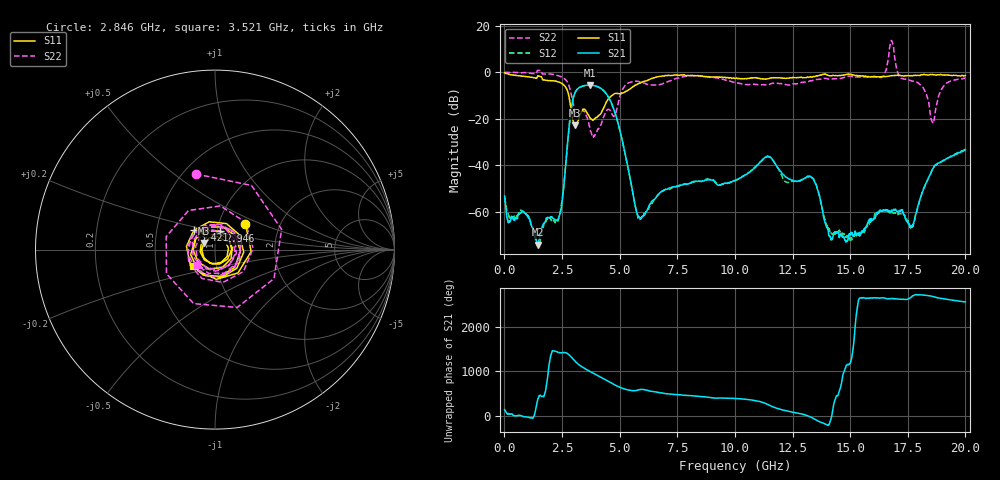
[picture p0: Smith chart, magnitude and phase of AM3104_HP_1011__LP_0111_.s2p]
!Created with skrf (http://scikit-rf.org).
# Hz S RI R 50.0
!freq ReS11 ImS11 ReS21 ImS21 ReS12 ImS12 ReS22 ImS22
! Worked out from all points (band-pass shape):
!   1601 points, 10 MHz to 20 GHz, reference 50 ohm
!   highest |S21| = -5.47 dB at 3.708 GHz (marker M1); lowest = -74.0 dB at 1.447 GHz (marker M2)
!   |S21| within 3 dB of the highest: 3.081 GHz to 4.359 GHz (1.277 GHz wide, 34.3 % of centre)
!   lowest |S11| = -22.8 dB at 3.046 GHz (marker M3), VSWR 1.16, Z = 44 + j3.32 ohm
!   |S11| at or under -10 dB: 2.794 GHz to 4.662 GHz (1.868 GHz wide, 50.1 % of centre)
!   |S22| runs from -28.1 to 13.6 dB; largest |S21 - S12| = 0.035
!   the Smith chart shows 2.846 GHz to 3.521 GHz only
!   S11 on the Smith chart (normalised r, x): 2.846 GHz: 1.34, +0.41; 2.946 GHz: 1.03, +0.22; 3.421 GHz: 0.77, +0.17; 3.521 GHz: 0.77, -0.14
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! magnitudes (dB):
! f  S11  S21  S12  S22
! 10 MHz  -0.3  -53.2  -53.8  0.0
! 1.447 GHz  -1.6  -74.0  -74.6  0.8
! 2.396 GHz  -4.3  -61.3  -61.6  -1.7
! 2.846 GHz  -13.0  -19.9  -19.9  -7.2
! 2.946 GHz  -19.5  -13.0  -13.0  -11.6
! 3.046 GHz  -22.8  -9.3  -9.3  -16.1
! 3.346 GHz  -16.9  -6.1  -6.2  -16.7
! 3.421 GHz  -16.0  -5.9  -5.9  -16.4
! 3.521 GHz  -16.4  -5.7  -5.7  -17.6
! 3.708 GHz  -19.4  -5.5  -5.5  -23.8
! 4.733 GHz  -9.5  -15.5  -15.5  -19.0
! 5.832 GHz  -4.9  -62.0  -63.3  -4.0
! 6.682 GHz  -1.9  -52.5  -52.4  -5.4
! 10.01 GHz  -2.7  -46.6  -46.6  -4.5
! 11.43 GHz  -2.8  -36.0  -36.2  -5.5
! 13.34 GHz  -2.1  -45.3  -45.2  -3.6
! 14.17 GHz  -1.5  -72.0  -68.9  -3.0
! 16.36 GHz  -1.9  -59.7  -59.6  -2.3
! 16.68 GHz  -1.6  -59.5  -59.8  7.2
! 17.68 GHz  -1.6  -66.1  -66.9  -3.8
! 18.58 GHz  -1.0  -41.7  -41.9  -21.5
! 20 GHz  -1.4  -33.4  -33.1  -2.5
